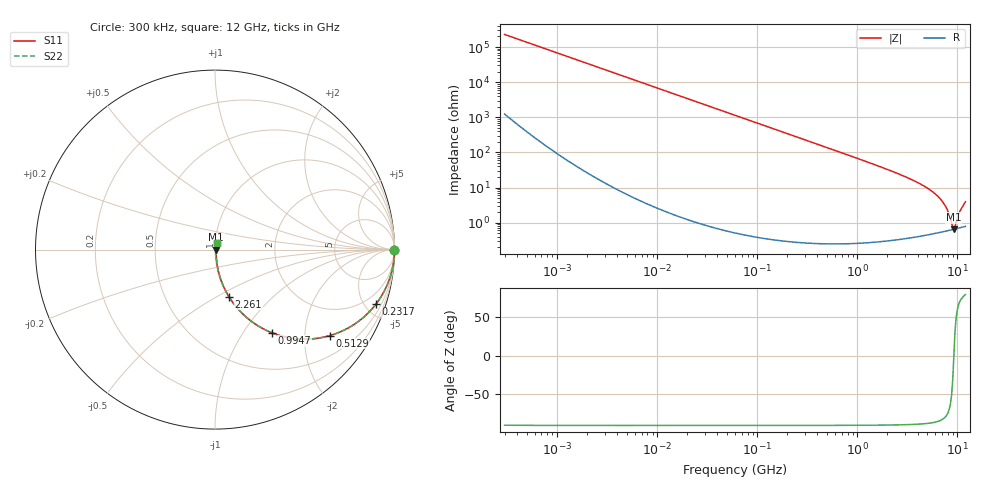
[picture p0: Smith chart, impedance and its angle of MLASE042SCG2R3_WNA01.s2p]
! MLASE042SCG2R3_WNA01  S-PARAMETER MODEL  ( General Type )
! Model Generated by TAIYO YUDEN Corporation (http://www.ty-top.com)
! Version 1.0
! TAIYO YUDEN Control No. 130801
! Copyright(c) 2013 TAIYO YUDEN CO.,LTD. All Rights Reserved.
! Product Description (link to TY-COMPAS)
! https://ds.yuden.co.jp/TYCOMPAS/or/detail?pn=MLASE042SCG2R3AWNA01&u=M
! Products Name : Multilayer Ceramic Capacitors
! Characteristics :
!  Capacitance : 2.3 pF , Rated Voltage : 16V , TCC : CG / C0G
!  Case Size : 0.4 x 0.2 / 0.016 x 0.008 [mm/inch] , Thickness : 0.2 / 0.008 [mm/inch]
!  (Conditions: Temperature = 25 degC , DC Bias Current/Voltage = 0A / 0V)
! External Node Assignments :
!  1  o---| |---o  2
! GND o---------o GND
! Frequency Range : 0.3MHz  -  12000MHz  [ 401 STEP ]
# MHz S RI R 50
! Freq[MHz].  S11 Real  S11 Imag  S21 Real  S21 Imag  S12 Real  S12 Imag  S22 Real  S22 Imag
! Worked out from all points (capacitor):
!   401 points, 300 kHz to 12 GHz, reference 50 ohm
!   read as one part in series: C = 2.32 pF near 316.3 kHz
!   lowest |Z| = 648 mohm at 9.207 GHz (marker M1)
!   series resonance near 9.201 GHz, so ESL is about 130 pH
!   S11 on the Smith chart (normalised r, x): 300 kHz: open; 231.7 MHz: 1.01, -5.91; 512.9 MHz: 1.00, -2.66; 994.7 MHz: 1.01, -1.36; 2.261 GHz: 1.01, -0.57; 12 GHz: 1.02, +0.08
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0.3  1 -0.000438  2.56e-06 0.000438  2.56e-06 0.000438  1 -0.000438
1.769972  1 -0.00258  8.85e-06 0.00258  8.85e-06 0.00258  1 -0.00258
10.44266  0.9998 -0.0152  0.000238 0.0152  0.000238 0.0152  0.9998 -0.0152
60  0.9923 -0.0869  0.00766 0.0869  0.00766 0.0869  0.9923 -0.0869
119.4772  0.9704 -0.1693  0.0296 0.1693  0.0296 0.1693  0.9704 -0.1693
231.6935  0.897 -0.3035  0.103 0.3035  0.103 0.3035  0.897 -0.3035
353.9943  0.7883 -0.4078  0.2117 0.4078  0.2117 0.4078  0.7883 -0.4078
512.9422  0.6389 -0.4794  0.3611 0.4794  0.3611 0.4794  0.6389 -0.4794
704.9044  0.4827 -0.4984  0.5173 0.4984  0.5173 0.4984  0.4827 -0.4984
994.7115  0.3171 -0.4635  0.6829 0.4635  0.6829 0.4635  0.3171 -0.4635
1441.349  0.1783 -0.3798  0.8217 0.3798  0.8217 0.3798  0.1783 -0.3798
2088.533  0.0905 -0.282  0.9095 0.282  0.9095 0.282  0.0905 -0.282
2261.293  0.0774 -0.2617  0.9226 0.2617  0.9226 0.2617  0.0774 -0.2617
4050.141  0.022 -0.1328  0.978 0.1328  0.978 0.1328  0.022 -0.1328
6026.253  0.00906 -0.064  0.9909 0.064  0.9909 0.064  0.00906 -0.064
7448.838  0.00659 -0.0313  0.9934 0.0313  0.9934 0.0313  0.00659 -0.0313
8064.993  0.00628 -0.0195  0.9937 0.0195  0.9937 0.0195  0.00628 -0.0195
8732.115  0.00627 -0.00773  0.9937 0.00773  0.9937 0.00773  0.00627 -0.00773
9207.246  0.00644 9.58e-05  0.9936 -9.58e-05  0.9936 -9.58e-05  0.00644 9.58e-05
9708.23  0.00674 0.00772  0.9933 -0.00772  0.9933 -0.00772  0.00674 0.00772
10793.46  0.00768 0.0221  0.9923 -0.0221  0.9923 -0.0221  0.00768 0.0221
12000  0.00923 0.038  0.9908 -0.038  0.9908 -0.038  0.00923 0.038
